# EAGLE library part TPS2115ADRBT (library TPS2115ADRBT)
Autoswitching Power Mux Source: Datasheet
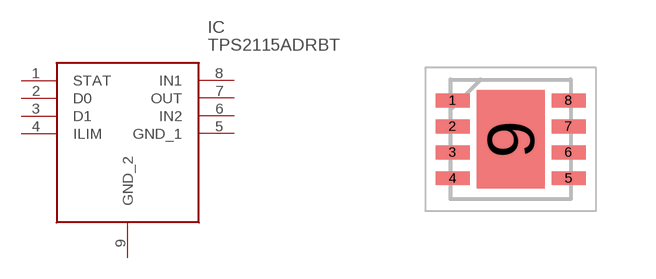
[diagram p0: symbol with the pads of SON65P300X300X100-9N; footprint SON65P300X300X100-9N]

Designator prefix IC

## TPS2115ADRBT (Arrow_Part_Number: TPS2115ADRBT; Arrow_Price-Stock: https://www.arrow.com/en/products/tps2115adrbt/texas-instruments.html?utm_currency=USD&region=nac; Description: Autoswitching Power Mux; Height: 1mm; Manufacturer_Name: Texas Instruments; Manufacturer_Part_Number: TPS2115ADRBT; Mouser_Part_Number: 595-TPS2115ADRBT; Mouser_Price-Stock: https://www.mouser.co.uk/ProductDetail/Texas-Instruments/TPS2115ADRBT?qs=g%2FrhRe7LVpRzfUPvVko3fA%3D%3D)  [SON65P300X300X100-9N]
1  STAT
2  D0
3  D1
4  ILIM
5  GND_1
6  IN2
7  OUT
8  IN1
9  GND_2

## Footprint SON65P300X300X100-9N (pad centres in mm)
DRB0008B
smd 0.85 x 0.35: 1 -1.45,0.975; 2 -1.45,0.325; 3 -1.45,-0.325; 4 -1.45,-0.975; 5 1.45,-0.975; 6 1.45,-0.325; 7 1.45,0.325; 8 1.45,0.975
smd 1.7 x 2.45: 9 0,0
